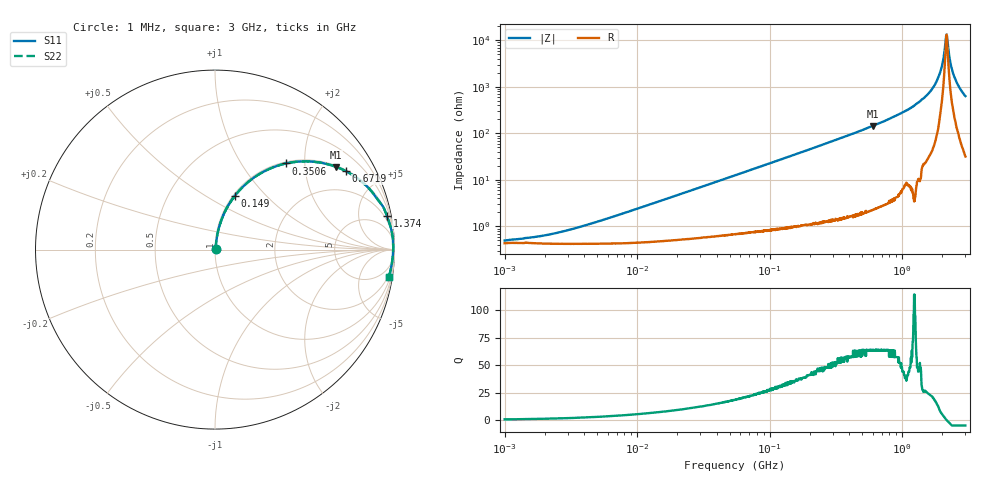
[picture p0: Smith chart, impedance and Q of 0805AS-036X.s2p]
!s-Parameter Generated by FASTRON Sdn. Bhd.
!FASTRON P/N : 0805AS-036X
!Keysight Technologies: E4991B_MY54100416_A.01.15
!Date: Mon Jun 15 12:50:14 2026
!Version  :Rev01  Mon Jun 15 12:50:14 2026
!Data & Calibration Information:
!Freq  S11  S21  S12  S22
!PortZ  Port1:50+j0  Port2:50+j0
!When reading reference impedance value at option line is always used.
! Remarks : This data is being provided solely for informational purposes.
# Hz S dB R 50
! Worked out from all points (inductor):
!   1601 points, 1 MHz to 3 GHz, reference 50 ohm
!   read as one part in series: L = 37.8 nH near 5.373 MHz
!   highest Q = 64 at 601.9 MHz (marker M1), where L = 38.4 nH
!   self-resonance near 2.156 GHz
!   S11 on the Smith chart (normalised r, x): 1 MHz: 1.01, +0.00; 149 MHz: 1.02, +0.68; 350.6 MHz: 1.03, +1.61; 671.9 MHz: 1.05, +3.30; 1.374 GHz: 1, +10; 3 GHz: 2, -13
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1000000  -46.10 28.7  -0.04 -0.1  -0.04 -0.1  -46.10 28.7
2014875  -43.80 48.1  -0.04 -0.3  -0.04 -0.3  -43.80 48.1
3804036  -40.00 64.5  -0.04 -0.5  -0.04 -0.5  -40.00 64.5
1.447069e7  -29.30 80.1  -0.05 -1.9  -0.05 -1.9  -29.30 80.1
5.504702e7  -18.10 79.8  -0.13 -7.1  -0.13 -7.1  -18.10 79.8
1.49005e8  -9.96 69.8  -0.55 -18.5  -0.55 -18.5  -9.96 69.8
2.083556e8  -7.45 63.6  -0.96 -25.1  -0.96 -25.1  -7.45 63.6
3.50605e8  -4.12 50.5  -2.25 -38.5  -2.25 -38.5  -4.12 50.5
6.018993e8  -1.75 34.3  -4.99 -54.8  -4.99 -54.8  -1.75 34.3
6.719458e8  -1.42 31.0  -5.77 -58.1  -5.77 -58.1  -1.42 31.0
7.925923e8  -1.00 26.1  -7.14 -63.0  -7.14 -63.0  -1.00 26.1
1.374365e9  -0.20 11.2  -14.20 -77.6  -14.20 -77.6  -0.20 11.2
1.621129e9  -0.12 7.2  -18.00 -80.3  -18.00 -80.3  -0.12 7.2
1.827992e9  -0.07 4.2  -22.70 -81.9  -22.70 -81.9  -0.07 4.2
1.970482e9  -0.06 2.3  -27.80 -78.8  -27.80 -78.8  -0.06 2.3
2.102926e9  -0.06 0.7  -37.10 -59.8  -37.10 -59.8  -0.06 0.7
2.156205e9  -0.06 0.1  -42.50 -10.6  -42.50 -10.6  -0.06 0.1
2.210833e9  -0.07 -0.5  -38.30 50.6  -38.30 50.6  -0.07 -0.5
2.347656e9  -0.07 -2.1  -28.70 75.5  -28.70 75.5  -0.07 -2.1
2.480502e9  -0.09 -3.5  -24.20 78.6  -24.20 78.6  -0.09 -3.5
2.714296e9  -0.12 -5.9  -19.70 79.5  -19.70 79.5  -0.12 -5.9
3e9  -0.17 -8.9  -16.20 78.2  -16.20 78.2  -0.17 -8.9
